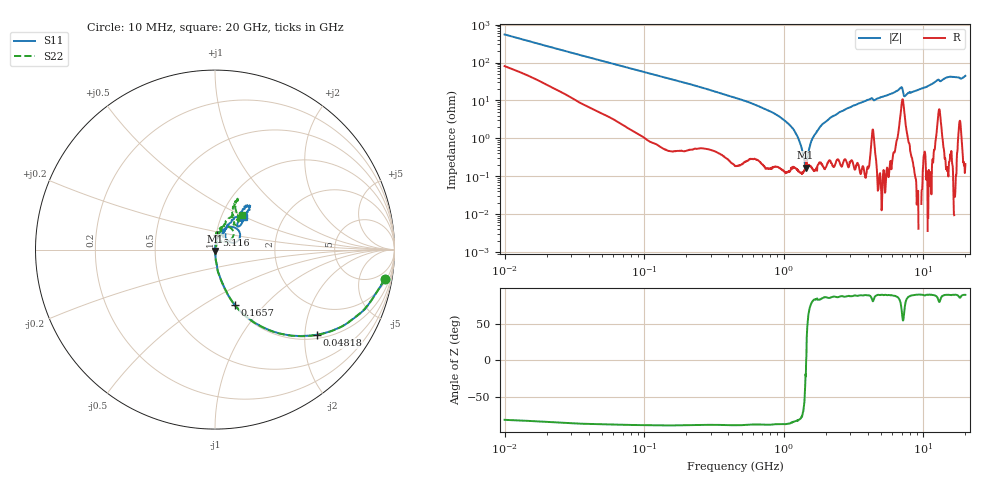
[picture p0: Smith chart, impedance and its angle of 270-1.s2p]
!Keysight Technologies,P5008B,MY61100088,A.16.20.02
!Date: Monday, May 27, 2024 17:38:18
!Correction: S11(C* 2-Port  )
!S21(C* 2-Port  )
!S12(C* 2-Port  )
!S22(C* 2-Port  )
!S2P File: Measurements: S11, S21, S12, S22:Log Frequency Sweep
# Hz S  dB  R 50
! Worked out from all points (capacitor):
!   1601 points, 10 MHz to 20 GHz, reference 50 ohm
!   read as one part in series: C = 29.3 pF near 10.39 MHz
!   lowest |Z| = 167 mohm at 1.432 GHz (marker M1)
!   series resonance near 1.446 GHz, so ESL is about 410 pH
!   S11 on the Smith chart (normalised r, x): 10 MHz: 2, -11; 48.18 MHz: 1.10, -2.30; 165.7 MHz: 1.01, -0.69; 5.116 GHz: 1.01, +0.17; 20 GHz: 1.28, +0.49
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1e7  -0.34 -9.9  -15.19 71.7  -15.20 71.7  -0.36 -9.9
3.555162e7  -1.72 -31.9  -5.50 55.0  -5.51 55.0  -1.73 -32.0
4.818375e7  -2.63 -40.0  -3.82 47.6  -3.82 47.6  -2.63 -40.1
1.263918e8  -7.77 -65.2  -0.85 24.1  -0.86 24.1  -7.76 -65.2
1.656983e8  -9.73 -70.4  -0.54 19.0  -0.54 19.0  -9.72 -70.4
4.472136e8  -18.48 -82.7  -0.08 6.6  -0.09 6.6  -18.48 -83.0
9.29478e8  -27.53 -85.6  -0.02 1.9  -0.03 1.9  -27.60 -85.8
1.173095e9  -32.98 -84.4  -0.01 0.7  -0.02 0.7  -32.91 -82.5
1.432139e9  -42.96 -80.1  -0.00 -0.3  -0.01 -0.4  -41.77 -64.7
1.523372e9  -52.96 -28.2  -0.00 -0.7  -0.01 -0.7  -46.87 -25.7
1.589917e9  -50.82 67.1  -0.00 -0.9  -0.01 -0.9  -47.51 20.8
1.850951e9  -37.26 80.7  -0.00 -1.7  -0.01 -1.7  -37.43 63.8
2.196181e9  -31.28 82.8  -0.00 -2.7  -0.01 -2.7  -31.70 73.5
3.846973e9  -23.09 87.9  -0.02 -7.0  -0.03 -7.0  -22.28 75.6
5.115731e9  -21.44 82.4  -0.02 -9.4  -0.03 -9.4  -21.31 76.1
5.652411e9  -20.21 77.3  -0.03 -10.7  -0.04 -10.7  -20.26 78.8
6.83533e9  -16.14 54.9  -0.36 -14.9  -0.37 -14.9  -16.75 66.3
7.480993e9  -21.35 43.3  -0.17 -11.4  -0.18 -11.4  -23.19 77.3
1.018741e10  -19.27 62.8  -0.05 -19.0  -0.07 -19.0  -19.47 71.5
1.489756e10  -10.47 53.9  -0.35 -28.9  -0.36 -28.9  -10.46 65.5
1.871311e10  -14.89 47.2  -0.19 -34.2  -0.20 -34.2  -15.12 53.6
2e10  -12.32 48.0  -0.21 -38.7  -0.22 -38.7  -12.24 51.3
